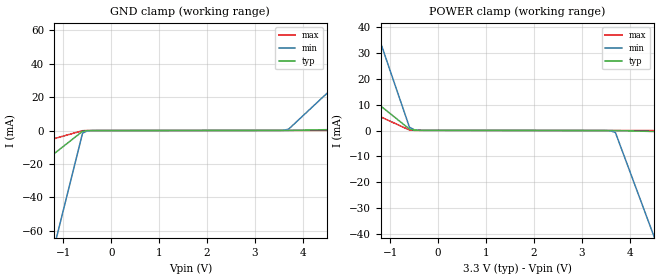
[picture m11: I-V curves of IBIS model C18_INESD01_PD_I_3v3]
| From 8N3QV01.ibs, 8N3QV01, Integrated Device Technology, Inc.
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[Model] C18_INESD01_PD_I_3v3
Model_type   Input
Polarity   Non-Inverting
Vinl = 0.8V
Vinh = 2.0V
|   typ   min   max
C_comp   2pF   1.5pF   2.5pF
|   typ   min   max
[Voltage range]   3.3V   3.135V   3.465V
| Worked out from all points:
|   GND clamp passes 1 mA (typ) near -0.62 V on its own axis
|   POWER clamp passes 1 mA (typ) near -0.63 V on its own axis
[GND_clamp]
|Voltage   I (typ)   I (min)   I (max)
-3.3V     -61.32mA   -311.6mA   -21.78mA
-1.2V     -13.98mA   -70.44mA   -4.913mA
-1.1V     -11.73mA   -58.96mA   -4.11mA
-600mV    -453.3uA   -1.545mA   -93.57uA
-500mV    -55.7uA    -216.7uA   -12.67uA
-400mV    -11.1uA    -31.44uA   -6.92uA
3.5V      69.96uA    87.78uA    59.56uA
3.7V      77.31uA    776.1uA    62.96uA
5.9V      1.265mA    59.68mA    100.6uA
6V        1.319mA    62.36mA    102.3uA
6.6V      1.643mA    78.42mA    112.6uA
[Power_clamp]
|Voltage   I (typ)   I (min)   I (max)
-3.3V     40.74mA    147.8mA    23.03mA
-3.2V     39.25mA    142.4mA    22.18mA
-1.4V     12.47mA    44.7mA     6.961mA
-1.3V     10.98mA    39.28mA    6.115mA
-600mV    567.9uA    1.285mA    195.9uA
-500mV    131.3uA    294.6uA    73.67uA
3.6V      -6.143uA   -107.8uA   -2.297uA
3.7V      -11.1uA    -783.3uA   -3.999uA
4.4V      -323.3uA   -35.71mA   -15.97uA
4.5V      -367.9uA   -40.7mA    -17.68uA
6.6V      -1.304mA   -145.5mA   -53.6uA
